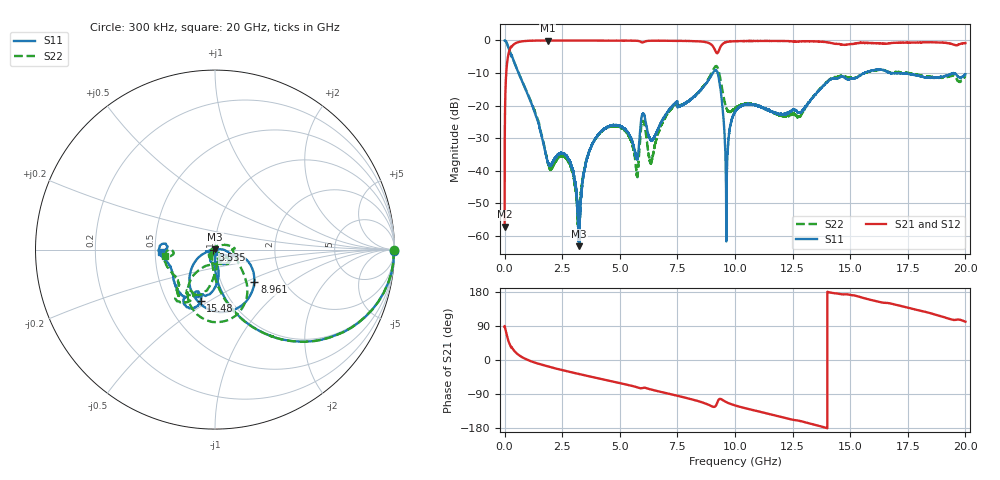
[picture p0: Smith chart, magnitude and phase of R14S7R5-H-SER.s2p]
!{R14S7R5}
!Johanson Technology Inc.
!www.johansontechnology.com
!Test Board Conditions:
!Substrate Type  RO4350B
!Substrate Thickness  20 mil
!Substrate Dk  3.66
!TL Type: GCPW
!TL Trace Width  36 mil
!TL Gap  12 mil
!Electrode orientation  Horizontal
!DUT TOPOLOGY	SERIES
!Mounting Pad LxW  26x36 mil
! Created Wed Nov 25 17:33:21 2020
! 2 Port Network Data from SP1.SP block
! freq  magS11  angS11  magS21  angS21  magS12  angS12  magS22  angS22
# khz S ma R 50
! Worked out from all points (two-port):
!   20001 points, 300 kHz to 20 GHz, reference 50 ohm
!   highest |S21| = -0.02 dB at 1.863 GHz (marker M1); lowest = -57.3 dB at 300 kHz (marker M2)
!   |S21| within 3 dB of the highest: 211.7 MHz to 9.137 GHz (8.925 GHz wide, 191 % of centre); 9.306 GHz to end of sweep
!   lowest |S11| = -63.2 dB at 3.228 GHz (marker M3), VSWR 1.00, Z = 50 + j0.0659 ohm
!   |S11| at or under -10 dB: 605.7 MHz to 9.041 GHz (8.435 GHz wide, 175 % of centre); 9.249 GHz to 15.62 GHz (6.372 GHz wide, 51.2 % of centre); 16.85 GHz to 19.48 GHz (2.628 GHz wide, 14.5 % of centre)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
!   |S22| runs from -60.8 to 0.0 dB; largest |S21 - S12| = 0.02
!   S11 on the Smith chart (normalised r, x): 300 kHz: open; 3.535 GHz: 0.97, -0.01; 8.961 GHz: 1.43, -0.57; 15.48 GHz: 0.73, -0.46; 20 GHz: 0.54, -0.01
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300  0.9961 -0.3  0.001372 88.1  0.001448 90.0  0.9966 -0.3
105300  0.895 -27.3  0.4427 62.6  0.4437 62.5  0.8945 -27.2
231300  0.6688 -49.7  0.7373 40.0  0.7389 39.9  0.67 -49.7
1863300  0.01398 -50.2  0.998 -16.8  0.9969 -16.8  0.01383 -151.5
2770300  0.01488 31.0  0.996 -30.5  0.9966 -30.5  0.0138 95.0
3228300  0.0006909 72.3  0.9964 -37.0  0.9962 -36.9  0.00126 -166.0
3334300  0.004539 -167.1  0.9963 -38.4  0.996 -38.4  0.005244 -109.6
3535300  0.01375 -163.5  0.9953 -41.2  0.996 -41.2  0.01412 -108.6
4515300  0.0475 -169.5  0.994 -54.5  0.9944 -54.4  0.04655 -118.7
5304300  0.04005 -165.9  0.9928 -65.1  0.9939 -65.1  0.03803 -136.0
5734300  0.01538 -114.0  0.9884 -71.6  0.9884 -71.7  0.008769 -114.1
5994300  0.07405 -88.8  0.9324 -73.7  0.9337 -73.6  0.05737 -91.6
6336300  0.02999 -92.2  0.9884 -77.5  0.9899 -77.5  0.01306 122.5
6667300  0.0442 -41.0  0.9918 -82.5  0.9905 -82.5  0.0378 41.3
8961300  0.2854 -39.7  0.8721 -121.3  0.8719 -121.3  0.3057 -53.8
9303300  0.2597 -121.3  0.7016 -103.8  0.7053 -103.8  0.3281 -116.0
9632300  0.003312 29.3  0.9466 -111.4  0.9478 -111.5  0.09074 -109.1
1.00003e7  0.07962 -12.4  0.9739 -119.7  0.9737 -119.8  0.09045 -62.2
1.33343e7  0.129 -81.1  0.9718 -169.0  0.9734 -169.0  0.1285 -89.5
1.54763e7  0.296 -105.5  0.9171 165.4  0.9225 165.2  0.2951 -115.0
1.66673e7  0.3175 -122.4  0.8991 150.1  0.8914 149.8  0.328 -129.6
2e7  0.3021 -177.7  0.9097 101.2  0.9087 101.5  0.281 -172.4
